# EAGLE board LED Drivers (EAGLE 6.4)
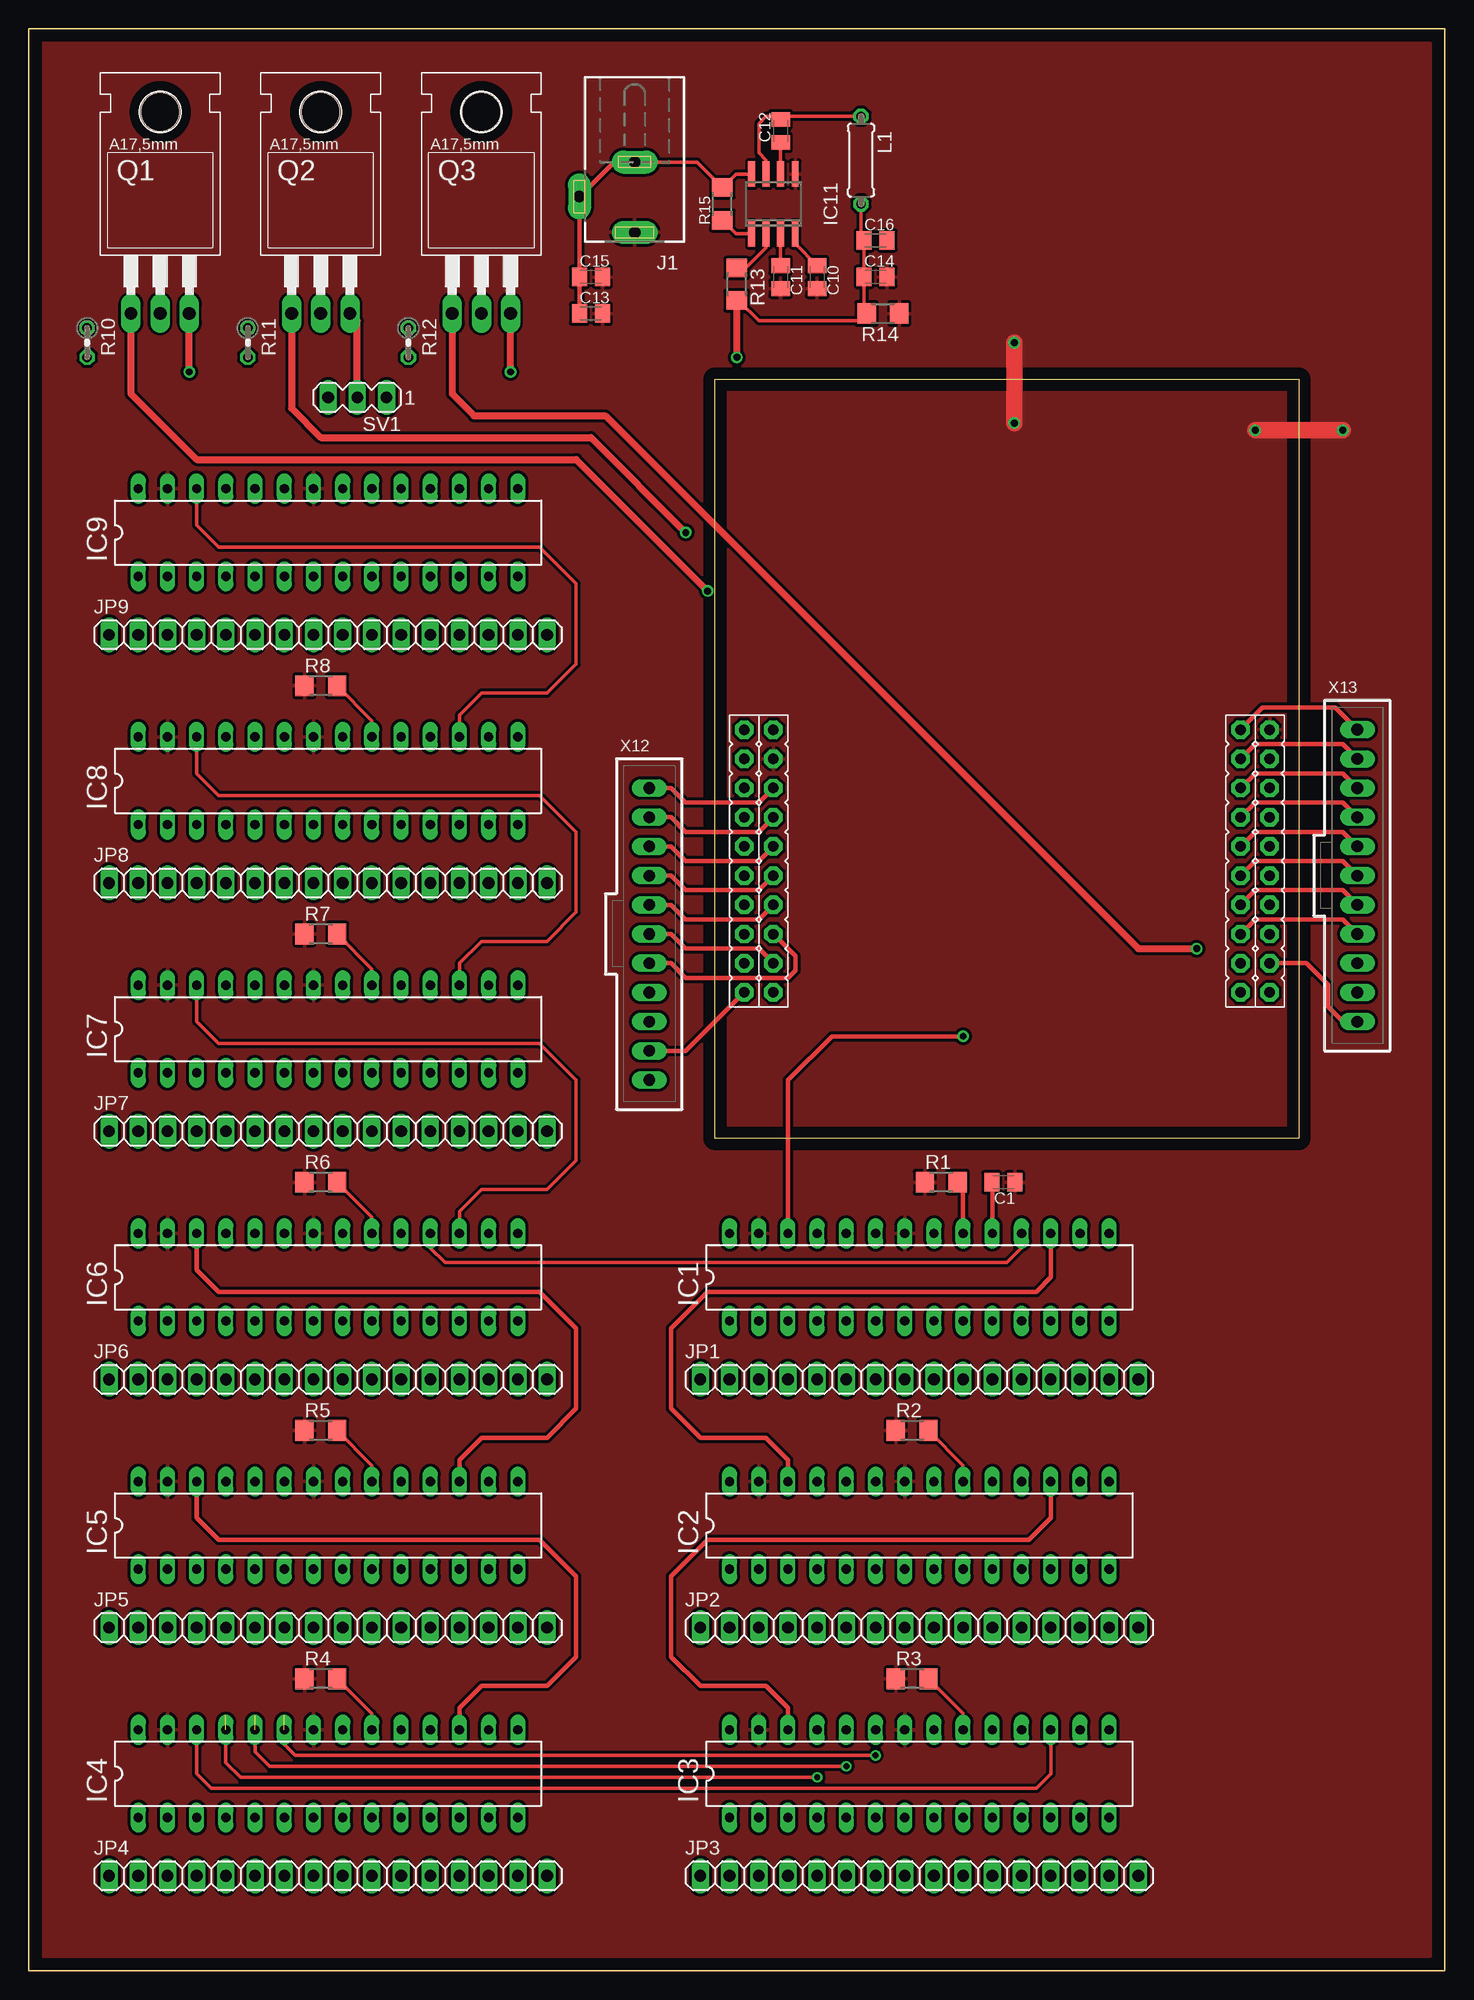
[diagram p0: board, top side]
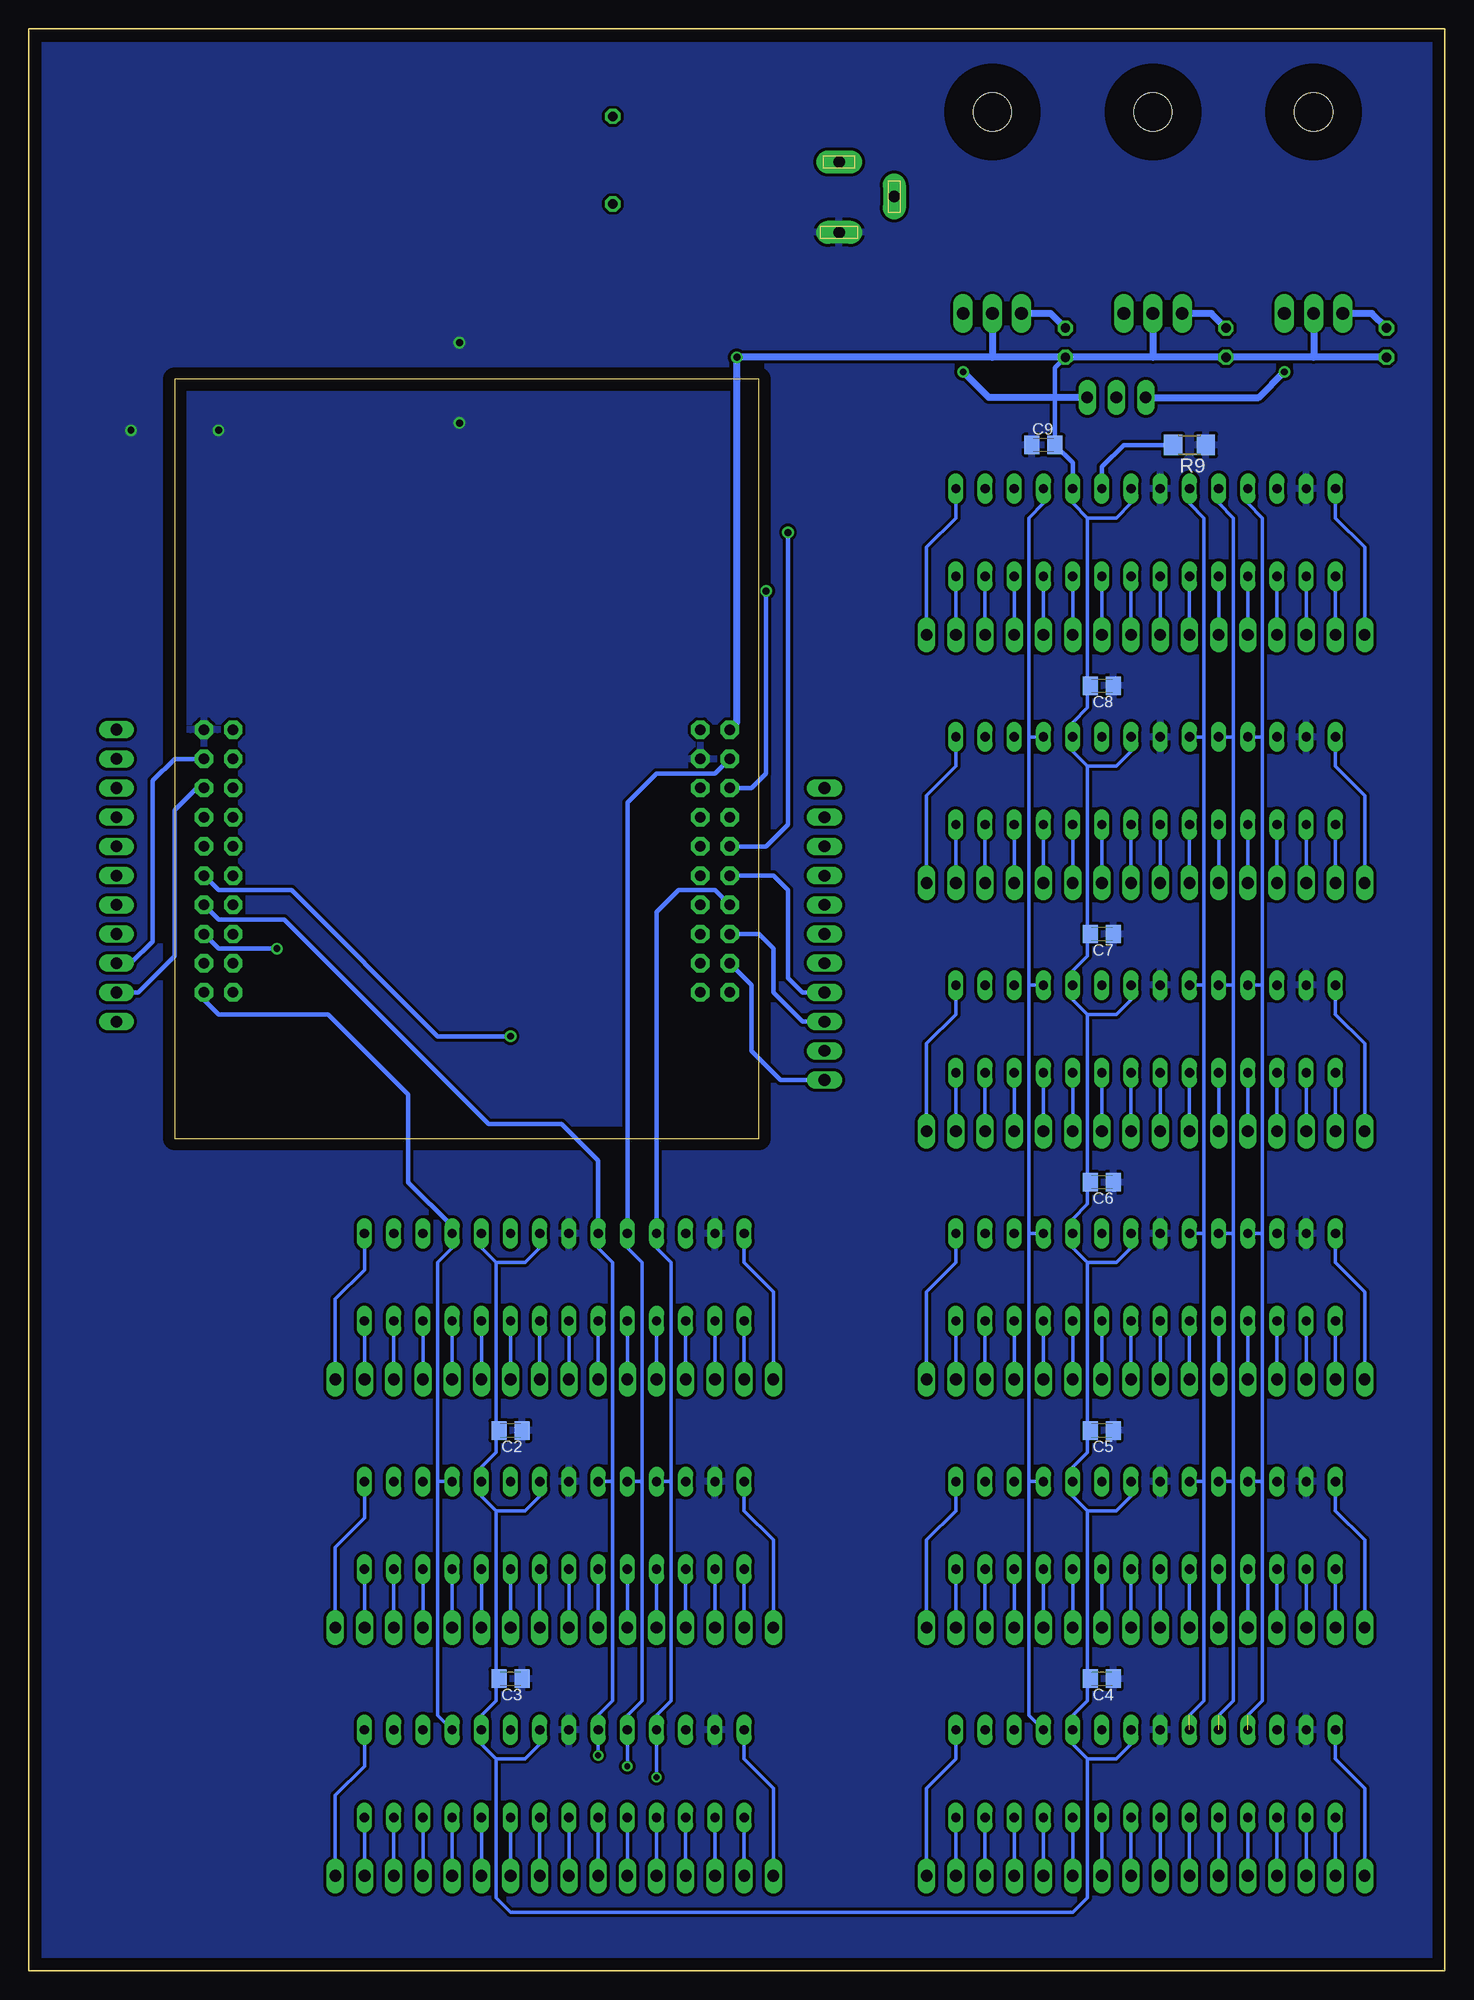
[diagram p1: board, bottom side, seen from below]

Size 123.19 x 168.91 mm. Coordinates in mm from the lower left corner, seen from the top.
Outline: 0,0 123.19,0 123.19,168.91 0,168.91 0,0
Copper layers (1*16): Top 0.035mm / dielectric 1.5mm / Bottom 0.035mm
Design rules "default *": minimum track width 10mil, minimum drill 24mil, track to track 10mil, track to pad 10mil, pad to pad 10mil, via to via 10mil, smd to smd 8mil, copper to edge 40mil, drill to drill 8mil, minimum pad ring 10mil, minimum via ring 8mil, stop-mask expansion 4mil, vias tented up to drill 0mil, thermal gap 10mil

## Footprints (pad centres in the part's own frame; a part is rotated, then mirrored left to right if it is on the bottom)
C0805K = smd 1.3 x 1.6: 1 -1,0; 2 1,0
DIP28 = drill 0.813 long: 1 -15.24,-3.81; 2 -12.7,-3.81; 3 -10.16,-3.81; 4 -7.62,-3.81; 5 -5.08,-3.81; 6 -2.54,-3.81; 7 0,-3.81; 8 2.54,-3.81; 9 5.08,-3.81; 10 7.62,-3.81; 11 10.16,-3.81; 12 12.7,-3.81; 13 15.24,-3.81; 14 17.78,-3.81; 15 17.78,3.81; 16 15.24,3.81; 17 12.7,3.81; 18 10.16,3.81; 19 7.62,3.81; 20 5.08,3.81; 21 2.54,3.81; 22 0,3.81; 23 -2.54,3.81; 24 -5.08,3.81; 25 -7.62,3.81; 26 -10.16,3.81; 27 -12.7,3.81; 28 -15.24,3.81
SOIC8 = smd 0.6 x 2.2: 1 -1.905,-2.6; 2 -0.635,-2.6; 3 0.635,-2.6; 4 1.905,-2.6; 5 1.905,2.6; 6 0.635,2.6; 7 -0.635,2.6; 8 -1.905,2.6
DCJ0202 = drill 1 pad 2 long: 1 0,3.1; 2 4.8,0; 3 0,-3
1X16 = drill 1.016 long: 1 -19.05,0; 2 -16.51,0; 3 -13.97,0; 4 -11.43,0; 5 -8.89,0; 6 -6.35,0; 7 -3.81,0; 8 -1.27,0; 9 1.27,0; 10 3.81,0; 11 6.35,0; 12 8.89,0; 13 11.43,0; 14 13.97,0; 15 16.51,0; 16 19.05,0
0207/7 = drill 0.813 octagon: 1 -3.81,0; 2 3.81,0
TO220 = drill 1.118 long: 1 -2.54,-6.35; 2 0,-6.35; 3 2.54,-6.35 | hole 3.302: 0,11.176
R1206 = smd 1.6 x 1.803: 1 -1.422,0; 2 1.422,0
0204V = drill 0.813 octagon: 1 -1.27,0; 2 1.27,0
MA03-1 = drill 1.016 long: 1 -2.54,0; 2 0,0; 3 2.54,0
LAUNCHPAD-XL = drill 0.914 pad 1.6 octagon: 3.3V 30.48,2.54; GND1 33.02,5.08; GND2 30.48,48.26; PA2 53.34,48.26; PA3 50.8,48.26; PA4 48.26,48.26; PA5 48.26,2.54; PA6 50.8,2.54; PA7 53.34,2.54; PB0 35.56,2.54; PB1 38.1,2.54; PB2 33.02,48.26; PB3 35.56,45.72; PB4 45.72,2.54; PB5 33.02,2.54; PB6 45.72,48.26; PB7 43.18,48.26; PC4 38.1,45.72; PC5 40.64,45.72; PC6 43.18,45.72; PC7 45.72,45.72; PD0 35.56,5.08; PD1 38.1,5.08; PD2 40.64,5.08; PD3 43.18,5.08; PD6 48.26,45.72; PD7 50.8,45.72; PE0 35.56,48.26; PE1 45.72,5.08; PE2 48.26,5.08; PE3 50.8,5.08; PE4 40.64,2.54; PE5 43.18,2.54; PF0 38.1,48.26; PF1 53.34,5.08; PF2 30.48,45.72; PF3 33.02,45.72; PF4 53.34,45.72; RST 40.64,48.26; VBUS 30.48,5.08
70543-11 = drill 1.016 long: 1 -12.7,0; 2 -10.16,0; 3 -7.62,0; 4 -5.08,0; 5 -2.54,0; 6 0,0; 7 2.54,0; 8 5.08,0; 9 7.62,0; 10 10.16,0; 11 12.7,0

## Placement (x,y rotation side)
C1  0.1uF  [C0805K]  84.77,68.58 180 top
C2  0.1uF  [C0805K]  81.28,46.99 180 bottom
C3  0.1uF  [C0805K]  81.28,25.4 180 bottom
C4  0.1uF  [C0805K]  29.84,25.4 180 bottom
C5  0.1uF  [C0805K]  29.84,46.99 180 bottom
C6  0.1uF  [C0805K]  29.84,68.58 180 bottom
C7  0.1uF  [C0805K]  29.84,90.17 180 bottom
C8  0.1uF  [C0805K]  29.84,111.76 180 bottom
C9  0.1uF  [C0805K]  34.92,132.72 0 bottom
C10  [C0805K]  68.58,147.32 270 top
C11  [C0805K]  65.41,147.32 270 top
C12  [C0805K]  65.41,160.02 90 top
C13  [C0805K]  48.9,144.15 0 top
C14  [C0805K]  73.66,147.32 0 top
C15  [C0805K]  48.9,147.32 0 top
C16  [C0805K]  73.66,150.5 0 top
IC1  [DIP28]  76.2,60.33 0 top
IC2  [DIP28]  76.2,38.73 0 top
IC3  [DIP28]  76.2,17.14 0 top
IC4  [DIP28]  24.77,17.14 0 top
IC5  [DIP28]  24.77,38.73 0 top
IC6  [DIP28]  24.77,60.33 0 top
IC7  [DIP28]  24.77,81.92 0 top
IC8  [DIP28]  24.77,103.5 0 top
IC9  [DIP28]  24.77,125.09 0 top
IC11  LT1257S  [SOIC8]  64.77,153.67 0 top
J1  DCJ0202  [DCJ0202]  52.7,154.31 180 top
JP1  [1X16]  77.47,51.44 0 top
JP2  [1X16]  77.47,29.84 0 top
JP3  [1X16]  77.47,8.26 0 top
JP4  [1X16]  26.04,8.26 0 top
JP5  [1X16]  26.04,29.84 0 top
JP6  [1X16]  26.04,51.44 0 top
JP7  [1X16]  26.04,73.03 0 top
JP8  [1X16]  26.04,94.61 0 top
JP9  [1X16]  26.04,116.2 0 top
L1  [0207/7]  72.39,157.48 270 top
Q1  BUZ171  [TO220]  11.43,150.5 0 top
Q2  BUZ171  [TO220]  25.4,150.5 0 top
Q3  BUZ171  [TO220]  39.37,150.5 0 top
R1  1.3K  [R1206]  79.38,68.58 0 top
R2  1.3K  [R1206]  76.83,46.99 0 top
R3  1.3K  [R1206]  76.83,25.4 0 top
R4  1.3K  [R1206]  25.4,25.4 0 top
R5  1.3K  [R1206]  25.4,46.99 0 top
R6  1.3K  [R1206]  25.4,68.58 0 top
R7  1.3K  [R1206]  25.4,90.17 0 top
R8  1.3K  [R1206]  25.4,111.76 0 top
R9  1.3K  [R1206]  22.23,132.72 180 bottom
R10  1K  [0204V]  5.08,141.6 270 top
R11  1K  [0204V]  19.05,141.6 270 top
R12  1K  [0204V]  33.02,141.6 270 top
R13  [R1206]  61.59,146.69 270 top
R14  [R1206]  74.3,144.15 180 top
R15  [R1206]  60.33,153.67 270 top
SV1  [MA03-1]  28.57,136.84 180 top
U$1  STELLARIS-LAUNCHPADSTELLARIS-LAUNCHPAD-XL  [LAUNCHPAD-XL]  59.69,138.43 270 top
X12  C-GRID-11-70543  [70543-11]  53.98,90.17 270 top
X13  C-GRID-11-70543  [70543-11]  115.57,95.25 270 top

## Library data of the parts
C1-C9 L1 = rcl
C10-C16 R1-R15 = resistor
IC1-IC9 = tcl5940(1)
IC11 = linear-technology; OC_FARNELL: unknown; OC_NEWARK: unknown
J1 = con-jack; OC_FARNELL: unknown; OC_NEWARK: unknown
JP1-JP9 = pinhead
Q1-Q3 = transistor-fet
SV1 = con-lstb; OC_FARNELL: unknown; OC_NEWARK: unknown
U$1 = StellarisLaunchPad_Fred
X12 X13 = con-molex; OC_FARNELL: unknown; OC_NEWARK: unknown

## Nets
+5V: C1.2 C2.2 C3.2 C4.2 C5.2 C6.2 C7.2 C8.2 C9.2 C14.1 C16.1 IC1.19 IC1.21 IC2.19 IC2.21 IC3.19 IC3.21 IC4.19 IC4.21 IC5.19 IC5.21 IC6.19 IC6.21 IC7.19 IC7.21 IC8.19 IC8.21 IC9.19 IC9.21 L1.2 Q1.2 Q2.2 Q3.2 R10.2 R11.2 R12.2 R13.2 R14.2 U$1.3.3V
GND: C1.1 C2.1 C3.1 C4.1 C5.1 C6.1 C7.1 C8.1 C9.1 C10.2 C11.2 C13.2 C14.2 C15.2 IC1.22 IC1.27 IC2.22 IC2.27 IC3.22 IC3.27 IC4.22 IC4.27 IC5.22 IC5.27 IC6.22 IC6.27 IC7.22 IC7.27 IC8.22 IC8.27 IC9.22 IC9.27 IC11.5 J1.1 R1.1 R2.1 R3.1 R4.1 R5.1 R6.1 R7.1 R8.1 R9.1 R14.1 U$1.GND1 U$1.GND2
N$1: IC1.17 IC2.26
N$2: IC1.20 R1.2
N$3: IC2.20 R2.2
N$4: IC2.28 JP2.1
N$5: IC2.3 JP2.4
N$6: IC2.4 JP2.5
N$7: IC2.5 JP2.6
N$8: IC2.6 JP2.7
N$9: IC2.7 JP2.8
N$10: IC2.8 JP2.9
N$11: IC2.9 JP2.10
N$12: IC2.10 JP2.11
N$13: IC2.11 JP2.12
N$14: IC2.12 JP2.13
N$15: IC1.28 JP1.1
N$16: IC2.13 JP2.14
N$17: IC2.14 JP2.15
N$18: IC2.15 JP2.16
N$19: IC1.1 JP1.2
N$20: IC1.2 JP1.3
N$21: IC1.3 JP1.4
N$22: IC1.4 JP1.5
N$23: IC1.5 JP1.6
N$24: IC1.6 JP1.7
N$25: IC1.7 JP1.8
N$26: IC1.8 JP1.9
N$27: IC1.9 JP1.10
N$28: IC1.10 JP1.11
N$29: IC1.11 JP1.12
N$30: IC1.12 JP1.13
N$31: IC1.13 JP1.14
N$32: IC1.14 JP1.15
N$33: IC1.15 JP1.16
N$34: IC2.1 JP2.2
N$35: IC2.2 JP2.3
N$36: IC2.17 IC3.26
N$37: IC3.20 R3.2
N$38: IC3.28 JP3.1
N$39: IC3.3 JP3.4
N$40: IC3.4 JP3.5
N$41: IC3.5 JP3.6
N$42: IC3.6 JP3.7
N$43: IC3.7 JP3.8
N$44: IC3.8 JP3.9
N$45: IC3.9 JP3.10
N$46: IC3.10 JP3.11
N$47: IC3.11 JP3.12
N$48: IC3.12 JP3.13
N$49: IC3.13 JP3.14
N$50: IC3.14 JP3.15
N$51: IC3.15 JP3.16
N$52: IC3.1 JP3.2
N$53: IC3.2 JP3.3
N$54: IC6.17 IC7.26
N$55: IC4.20 R4.2
N$56: IC4.28 JP4.1
N$57: IC4.3 JP4.4
N$58: IC4.4 JP4.5
N$59: IC4.5 JP4.6
N$60: IC4.6 JP4.7
N$61: IC4.7 JP4.8
N$62: IC4.8 JP4.9
N$63: IC4.9 JP4.10
N$64: IC4.10 JP4.11
N$65: IC4.11 JP4.12
N$66: IC4.12 JP4.13
N$67: IC4.13 JP4.14
N$68: IC4.14 JP4.15
N$69: IC4.15 JP4.16
N$70: IC4.1 JP4.2
N$71: IC4.2 JP4.3
N$72: IC4.17 IC5.26
N$73: IC5.20 R5.2
N$74: IC5.28 JP5.1
N$75: IC5.3 JP5.4
N$76: IC5.4 JP5.5
N$77: IC5.5 JP5.6
N$78: IC5.6 JP5.7
N$79: IC5.7 JP5.8
N$80: IC5.8 JP5.9
N$81: IC5.9 JP5.10
N$82: IC5.10 JP5.11
N$83: IC5.11 JP5.12
N$84: IC5.12 JP5.13
N$85: IC5.13 JP5.14
N$86: IC5.14 JP5.15
N$87: IC5.15 JP5.16
N$88: IC5.1 JP5.2
N$89: IC5.2 JP5.3
N$90: IC5.17 IC6.26
N$91: IC6.20 R6.2
N$92: IC6.28 JP6.1
N$93: IC6.3 JP6.4
N$94: IC6.4 JP6.5
N$95: IC6.5 JP6.6
N$96: IC6.6 JP6.7
N$97: IC6.7 JP6.8
N$98: IC6.8 JP6.9
N$99: IC6.9 JP6.10
N$100: IC6.10 JP6.11
N$101: IC6.11 JP6.12
N$102: IC6.12 JP6.13
N$103: IC6.13 JP6.14
N$104: IC6.14 JP6.15
N$105: IC6.15 JP6.16
N$106: IC6.1 JP6.2
N$107: IC6.2 JP6.3
N$108: IC1.25 IC2.25 IC3.25 IC4.25 IC5.25 IC6.25 IC7.25 IC8.25 IC9.25 U$1.PB4
N$109: IC7.20 R7.2
N$110: IC7.28 JP7.1
N$111: IC7.3 JP7.4
N$112: IC7.4 JP7.5
N$113: IC7.5 JP7.6
N$114: IC7.6 JP7.7
N$115: IC7.7 JP7.8
N$116: IC7.8 JP7.9
N$117: IC7.9 JP7.10
N$118: IC7.10 JP7.11
N$119: IC7.11 JP7.12
N$120: IC7.12 JP7.13
N$121: IC7.13 JP7.14
N$122: IC7.14 JP7.15
N$123: IC7.15 JP7.16
N$124: IC7.1 JP7.2
N$125: IC7.2 JP7.3
N$126: IC1.18 IC2.18 IC3.18 IC4.18 IC5.18 IC6.18 IC7.18 IC8.18 IC9.18 U$1.PA2
N$127: IC8.20 R8.2
N$128: IC8.28 JP8.1
N$129: IC8.3 JP8.4
N$130: IC8.4 JP8.5
N$131: IC8.5 JP8.6
N$132: IC8.6 JP8.7
N$133: IC8.7 JP8.8
N$134: IC8.8 JP8.9
N$135: IC8.9 JP8.10
N$136: IC8.10 JP8.11
N$137: IC8.11 JP8.12
N$138: IC8.12 JP8.13
N$139: IC8.13 JP8.14
N$140: IC8.14 JP8.15
N$141: IC8.15 JP8.16
N$142: IC8.1 JP8.2
N$143: IC8.2 JP8.3
N$144: IC8.17 IC9.26
N$145: IC9.20 R9.2
N$146: IC9.28 JP9.1
N$147: IC9.3 JP9.4
N$148: IC9.4 JP9.5
N$149: IC9.5 JP9.6
N$150: IC9.6 JP9.7
N$151: IC9.7 JP9.8
N$152: IC9.8 JP9.9
N$153: IC9.9 JP9.10
N$154: IC9.10 JP9.11
N$155: IC9.11 JP9.12
N$156: IC9.12 JP9.13
N$157: IC9.13 JP9.14
N$158: IC9.14 JP9.15
N$159: IC9.15 JP9.16
N$160: IC9.1 JP9.2
N$161: IC9.2 JP9.3
N$162: IC11.1 R15.2
N$163: IC1.26 U$1.PB7
N$164: U$1.PE1 X12.5
N$165: U$1.PF3 X13.2
N$166: U$1.PF2 X13.1
N$167: U$1.PB3 X13.3
N$168: U$1.PC4 X13.4
N$169: U$1.PC5 X13.5
N$170: U$1.PC6 X13.6
N$171: U$1.PC7 X13.7
N$172: U$1.PD6 X13.8
N$173: U$1.PB2 X13.9
N$174: U$1.PE0 X13.10
N$175: U$1.PA3 X13.11
N$176: Q3.1 R12.1 U$1.PA4
N$177: Q2.1 R11.1 U$1.PE4
N$178: U$1.PD0 X12.1
N$179: U$1.PD1 X12.2
N$180: U$1.PD2 X12.3
N$181: U$1.PD3 X12.4
N$182: IC1.23 IC2.23 IC3.23 IC4.23 IC5.23 IC6.23 IC7.23 IC8.23 IC9.23 U$1.PB6
N$183: U$1.PE3 X12.6
N$184: U$1.PE2 X12.7
N$185: U$1.PE5 X12.8
N$186: U$1.PA5 X12.9
N$187: U$1.PA7 X12.10
N$188: U$1.PA6 X12.11
N$189: IC1.24 IC2.24 IC3.24 IC4.24 IC5.24 IC6.24 IC7.24 IC8.24 IC9.24 U$1.PB5
N$190: Q1.3 SV1.3
N$191: Q2.3 SV1.2
N$192: Q3.3 SV1.1
N$193: Q1.1 R10.1 U$1.PB0
N$194: C13.1 C15.1 IC11.8 J1.2 J1.3 R15.1
N$195: C11.1 IC11.3
N$197: C10.1 IC11.4
N$198: C12.1 IC11.6
N$199: C12.2 IC11.7 L1.1
N$200: IC11.2 R13.1
N$202: IC3.17 IC4.26
N$204: IC7.17 IC8.26
RST: U$1.RST
VBUS: U$1.VBUS

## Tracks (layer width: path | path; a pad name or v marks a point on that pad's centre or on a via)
+5V  (via drill 0.6)
  Top 0.305: L1.2 72.39,150.76 C16.1 C14.1 72.66,144.36 R14.2 72.24,143.51 63.5,143.51 61.75,145.26 R13.2 61.59,144.78
  Top 0.406: IC1.19 83.82,68.53 C1.2
  Top 0.61: v61.59,140.34 R13.2
  Bottom 0.305: IC4.21 27.3,19.68 28.57,18.41 31.11,18.41 | 31.11,126.36 32.38,127.64 IC9.19 | IC9.21 27.3,127.64 28.57,126.36 31.11,126.36 | 31.11,104.78 32.38,106.05 IC8.19 32.38,108.58 31.11,109.86 31.11,111.49 C8.2 31.11,112.03 31.11,126.36 | IC8.21 27.3,106.05 28.57,104.78 31.11,104.78 | 31.11,83.19 32.38,84.45 IC7.19 32.38,87 31.11,88.27 31.11,89.9 C7.2 31.11,90.44 31.11,104.78 | IC7.21 27.3,84.45 28.57,83.19 31.11,83.19 | 31.11,61.59 32.38,62.87 IC6.19 32.38,65.41 31.11,66.67 31.11,68.31 C6.2 31.11,68.85 31.11,83.19 | IC6.21 27.3,62.87 28.57,61.59 31.11,61.59 | 31.11,40.01 32.38,41.27 IC5.19 32.38,43.81 31.11,45.09 31.11,46.62 | 31.11,18.41 32.38,19.68 IC4.19 32.38,22.23 31.11,23.5 31.11,25.13 C4.2 31.11,25.67 31.11,40.01 | IC5.21 27.3,41.27 28.57,40.01 31.11,40.01 | IC3.21 78.74,19.68 80.01,18.41 82.55,18.41 | 82.55,40.01 83.82,41.27 IC2.19 83.82,43.81 82.55,45.09 82.55,46.72 | IC2.21 78.74,41.27 80.01,40.01 82.55,40.01 | 82.55,61.59 83.82,62.87 IC1.19 | IC1.21 78.74,62.87 80.01,61.59 82.55,61.59 | 82.55,18.41 83.82,19.68 IC3.19 83.82,22.23 82.55,23.5 82.55,25.13 C3.2 82.55,25.67 82.55,40.01 | 82.55,18.41 82.55,6.35 81.28,5.08 32.38,5.08 31.11,6.35 31.11,18.41 | 82.55,46.72 C2.2 | 82.55,61.59 82.55,46.72 | 31.11,46.72 C5.2 31.11,46.62 | 31.11,61.59 31.11,46.72 | 31.11,46.72 31.11,46.62
  Bottom 0.406: IC9.19 32.38,131.18 C9.2 33.92,139.43 R12.2
  Bottom 0.61: R10.2 11.43,140.34 | 11.43,140.34 R11.2 25.4,140.34 | 25.4,140.34 R12.2 39.37,140.34 | Q1.2 11.43,140.34 | Q2.2 25.4,140.34 | 39.37,140.34 v61.59,140.34 61.59,108.58 U$1.3.3V | Q3.2 39.37,140.34
GND  (via drill 0.6)
  Top 1.422: v85.72,141.6 v85.72,134.62 | v114.3,133.99 v106.68,133.99
  pour Bottom: 1.27,1.27 121.92,1.27 121.92,167.64 1.27,167.64
  pour Top: 1.27,1.27 121.92,1.27 121.92,167.64 1.27,167.64
N$1
  Top 0.406: IC1.17 88.9,60.33 87.63,59.05 59.05,59.05 55.88,55.88 55.88,48.9 58.42,46.35 64.14,46.35 66.04,44.45 IC2.26
N$2
  Top 0.406: IC1.20 81.28,68.1 R1.2
N$3
  Top 0.305: IC2.20 81.28,43.97 R2.2
N$4
  Bottom 0.305: IC2.28 60.96,40.01 58.42,37.47 JP2.1
N$5
  Bottom 0.305: IC2.3 JP2.4
N$6
  Bottom 0.305: IC2.4 JP2.5
N$7
  Bottom 0.305: IC2.5 JP2.6
N$8
  Bottom 0.305: IC2.6 JP2.7
N$9
  Bottom 0.305: IC2.7 JP2.8
N$10
  Bottom 0.305: JP2.9 IC2.8
N$11
  Bottom 0.305: IC2.9 JP2.10
N$12
  Bottom 0.305: IC2.10 JP2.11
N$13
  Bottom 0.305: IC2.11 JP2.12
N$14
  Bottom 0.305: IC2.12 JP2.13
N$15
  Bottom 0.305: IC1.28 60.96,61.59 58.42,59.05 JP1.1
N$16
  Bottom 0.305: IC2.13 JP2.14
N$17
  Bottom 0.305: IC2.14 JP2.15
N$18
  Bottom 0.305: IC2.15 93.98,39.37 96.52,36.83 JP2.16
N$19
  Bottom 0.305: IC1.1 JP1.2
N$20
  Bottom 0.305: IC1.2 JP1.3
N$21
  Bottom 0.305: IC1.3 JP1.4
N$22
  Bottom 0.305: IC1.4 JP1.5
N$23
  Bottom 0.305: IC1.5 JP1.6
N$24
  Bottom 0.305: IC1.6 JP1.7
N$25
  Bottom 0.305: IC1.7 JP1.8
N$26
  Bottom 0.305: IC1.8 JP1.9
N$27
  Bottom 0.305: IC1.9 JP1.10
N$28
  Bottom 0.305: IC1.10 JP1.11
N$29
  Bottom 0.305: IC1.11 JP1.12
N$30
  Bottom 0.305: IC1.12 JP1.13
N$31
  Bottom 0.305: IC1.13 JP1.14
N$32
  Bottom 0.305: IC1.14 JP1.15
N$33
  Bottom 0.305: IC1.15 93.98,60.96 96.52,58.42 JP1.16
N$34
  Bottom 0.305: IC2.1 JP2.2
N$35
  Bottom 0.305: JP2.3 IC2.2
N$36
  Top 0.406: IC2.17 88.9,39.37 87,37.47 59.05,37.47 55.88,34.29 55.88,27.3 58.42,24.77 64.14,24.77 66.04,22.86 IC3.26
N$37
  Top 0.305: IC3.20 81.28,22.38 R3.2
N$38
  Bottom 0.305: IC3.28 60.96,18.41 58.42,15.88 JP3.1
N$39
  Bottom 0.305: IC3.3 JP3.4
N$40
  Bottom 0.305: IC3.4 JP3.5
N$41
  Bottom 0.305: IC3.5 JP3.6
N$42
  Bottom 0.305: IC3.6 JP3.7
N$43
  Bottom 0.305: IC3.7 JP3.8
N$44
  Bottom 0.305: IC3.8 JP3.9
N$45
  Bottom 0.305: IC3.9 JP3.10
N$46
  Bottom 0.305: IC3.10 JP3.11
N$47
  Bottom 0.305: IC3.11 JP3.12
N$48
  Bottom 0.305: IC3.12 JP3.13
N$49
  Bottom 0.305: IC3.13 JP3.14
N$50
  Bottom 0.305: IC3.14 JP3.15
N$51
  Bottom 0.305: IC3.15 93.98,17.78 96.52,15.24 JP3.16
N$52
  Bottom 0.305: IC3.1 JP3.2
N$53
  Bottom 0.305: IC3.2 JP3.3
N$54
  Top 0.305: IC6.17 37.47,66.04 39.37,67.94 45.09,67.94 47.62,70.48 47.62,77.47 44.45,80.64 16.51,80.64 14.61,82.55 IC7.26
N$55
  Top 0.305: IC4.20 29.84,22.38 R4.2
N$56
  Bottom 0.305: JP4.1 6.99,15.88 9.53,18.41 IC4.28
N$57
  Bottom 0.305: JP4.4 IC4.3
N$58
  Bottom 0.305: IC4.4 JP4.5
N$59
  Bottom 0.305: JP4.6 IC4.5
N$60
  Bottom 0.305: IC4.6 JP4.7
N$61
  Bottom 0.305: JP4.8 IC4.7
N$62
  Bottom 0.305: IC4.8 JP4.9
N$63
  Bottom 0.305: JP4.10 IC4.9
N$64
  Bottom 0.305: IC4.10 JP4.11
N$65
  Bottom 0.305: JP4.12 IC4.11
N$66
  Bottom 0.305: IC4.12 JP4.13
N$67
  Bottom 0.305: JP4.14 IC4.13
N$68
  Bottom 0.305: IC4.14 JP4.15
N$69
  Bottom 0.305: IC4.15 42.55,18.41 45.09,15.88 JP4.16
N$70
  Bottom 0.305: JP4.2 IC4.1
N$71
  Bottom 0.305: IC4.2 JP4.3
N$72
  Top 0.406: IC4.17 37.47,22.86 39.37,24.77 45.09,24.77 47.62,27.3 47.62,34.29 44.45,37.47 16.51,37.47 14.61,39.37 IC5.26
N$73
  Top 0.305: IC5.20 29.84,43.97 R5.2
N$74
  Bottom 0.305: IC5.28 9.53,40.01 6.99,37.47 JP5.1
N$75
  Bottom 0.305: JP5.4 IC5.3
N$76
  Bottom 0.305: JP5.5 IC5.4
N$77
  Bottom 0.305: IC5.5 JP5.6
N$78
  Bottom 0.305: JP5.7 IC5.6
N$79
  Bottom 0.305: IC5.7 JP5.8
N$80
  Bottom 0.305: JP5.9 IC5.8
N$81
  Bottom 0.305: IC5.9 JP5.10
N$82
  Bottom 0.305: JP5.11 IC5.10
N$83
  Bottom 0.305: IC5.11 JP5.12
N$84
  Bottom 0.305: JP5.13 IC5.12
N$85
  Bottom 0.305: IC5.13 JP5.14
N$86
  Bottom 0.305: JP5.15 IC5.14
N$87
  Bottom 0.305: IC5.15 42.55,40.01 45.09,37.47 JP5.16
N$88
  Bottom 0.305: JP5.2 IC5.1
N$89
  Bottom 0.305: IC5.2 JP5.3
N$90
  Top 0.406: IC5.17 37.47,44.45 39.37,46.35 45.09,46.35 47.62,48.9 47.62,55.88 44.45,59.05 16.51,59.05 14.61,60.96 IC6.26
N$91
  Top 0.305: IC6.20 29.84,65.56 R6.2
N$92
  Bottom 0.305: IC6.28 9.53,61.59 6.99,59.05 JP6.1
N$93
  Bottom 0.305: IC6.3 JP6.4
N$94
  Bottom 0.305: IC6.4 JP6.5
N$95
  Bottom 0.305: IC6.5 JP6.6
N$96
  Bottom 0.305: IC6.6 JP6.7
N$97
  Bottom 0.305: IC6.7 JP6.8
N$98
  Bottom 0.305: IC6.8 JP6.9
N$99
  Bottom 0.305: IC6.9 JP6.10
N$100
  Bottom 0.305: IC6.10 JP6.11
N$101
  Bottom 0.305: IC6.11 JP6.12
N$102
  Bottom 0.305: JP6.13 IC6.12
N$103
  Bottom 0.305: IC6.13 JP6.14
N$104
  Bottom 0.305: JP6.15 IC6.14
N$105
  Bottom 0.305: IC6.15 42.55,61.59 45.09,59.05 JP6.16
N$106
  Bottom 0.305: IC6.1 JP6.2
N$107
  Bottom 0.305: IC6.2 JP6.3
N$108  (via drill 0.5)  (1 unrouted)
  Top 0.305: IC4.25 17.14,18.1 18.41,16.83 v68.58,16.83
  Bottom 0.305: 17.14,22.23 15.88,23.5 15.88,42.55 | 15.88,42.55 15.88,64.14 | 15.88,64.14 15.88,85.72 | 15.88,85.72 15.88,107.31 | 15.88,107.31 15.88,126.36 17.14,127.64 IC9.25 | IC8.25 15.88,107.31 | IC6.25 15.88,64.14 | IC5.25 15.88,42.55 | IC1.25 68.58,62.87 67.31,61.59 67.31,42.55 | 67.31,42.55 67.31,23.5 68.58,22.23 IC3.25 v68.58,16.83 | IC2.25 67.31,42.55 | IC7.25 15.88,85.72
  Bottom 0.406: IC1.25 68.58,92.08 66.67,93.98 63.5,93.98 U$1.PB4
N$109
  Top 0.305: IC7.20 29.84,87.15 R7.2
N$110
  Bottom 0.305: JP7.1 6.99,80.64 9.53,83.19 IC7.28
N$111
  Bottom 0.305: IC7.3 JP7.4
N$112
  Bottom 0.305: IC7.4 JP7.5
N$113
  Bottom 0.305: IC7.5 JP7.6
N$114
  Bottom 0.305: IC7.6 JP7.7
N$115
  Bottom 0.305: IC7.7 JP7.8
N$116
  Bottom 0.305: JP7.9 IC7.8
N$117
  Bottom 0.305: IC7.9 JP7.10
N$118
  Bottom 0.305: JP7.11 IC7.10
N$119
  Bottom 0.305: JP7.12 IC7.11
N$120
  Bottom 0.305: JP7.13 IC7.12
N$121
  Bottom 0.305: JP7.14 IC7.13
N$122
  Bottom 0.305: JP7.15 IC7.14
N$123
  Bottom 0.305: IC7.15 42.55,83.19 45.09,80.64 JP7.16
N$124
  Bottom 0.305: JP7.2 IC7.1
N$125
  Bottom 0.305: IC7.2 JP7.3
N$126
  Top 0.305: IC1.18 86.36,62.87 85.09,61.59 36.2,61.59 34.92,62.87 IC6.18
  Bottom 0.305: IC1.18 86.36,62.87 87.63,61.59 87.63,42.55 | 87.63,42.55 87.63,22.23 IC3.18 | IC2.18 87.63,42.55 | IC4.18 36.2,22.23 36.2,42.55 | 36.2,42.55 36.2,64.14 | 36.2,64.14 36.2,85.72 | 36.2,85.72 IC7.18 | IC6.18 36.2,64.14 | IC5.18 36.2,42.55 | IC9.18 34.92,127.64 36.2,126.36 36.2,107.31 | 36.2,107.31 36.2,85.72 | IC8.18 36.2,107.31
  Bottom 0.406: U$1.PA2 107.95,84.45 106.68,83.19 97.16,83.19 90.17,76.2 90.17,68.58 86.36,64.77 IC1.18
N$127
  Top 0.305: IC8.20 29.84,108.74 R8.2
N$128
  Bottom 0.305: IC8.28 9.53,104.78 6.99,102.23 JP8.1
N$129
  Bottom 0.305: IC8.3 JP8.4
N$130
  Bottom 0.305: IC8.4 JP8.5
N$131
  Bottom 0.305: IC8.5 JP8.6
N$132
  Bottom 0.305: JP8.7 IC8.6
N$133
  Bottom 0.305: JP8.8 IC8.7
N$134
  Bottom 0.305: IC8.8 JP8.9
N$135
  Bottom 0.305: JP8.10 IC8.9
N$136
  Bottom 0.305: IC8.10 JP8.11
N$137
  Bottom 0.305: JP8.12 IC8.11
N$138
  Bottom 0.305: IC8.12 JP8.13
N$139
  Bottom 0.305: JP8.14 IC8.13
N$140
  Bottom 0.305: IC8.14 JP8.15
N$141
  Bottom 0.305: IC8.15 42.55,104.78 45.09,102.23 JP8.16
N$142
  Bottom 0.305: JP8.2 IC8.1
N$143
  Bottom 0.305: JP8.3 IC8.2
N$144
  Top 0.305: IC8.17 37.47,109.22 39.37,111.12 45.09,111.12 47.62,113.67 47.62,120.65 44.45,123.83 16.51,123.83 14.61,125.73 IC9.26
N$145
  Bottom 0.406: IC9.20 29.84,130.81 27.94,132.72 R9.2
N$146
  Bottom 0.305: IC9.28 9.53,126.36 6.99,123.83 JP9.1
N$147
  Bottom 0.305: JP9.4 IC9.3
N$148
  Bottom 0.305: IC9.4 JP9.5
N$149
  Bottom 0.305: JP9.6 IC9.5
N$150
  Bottom 0.305: IC9.6 JP9.7
N$151
  Bottom 0.305: JP9.8 IC9.7
N$152
  Bottom 0.305: IC9.8 JP9.9
N$153
  Bottom 0.305: JP9.10 IC9.9
N$154
  Bottom 0.305: IC9.10 JP9.11
N$155
  Bottom 0.305: JP9.12 IC9.11
N$156
  Bottom 0.305: IC9.12 JP9.13
N$157
  Bottom 0.305: JP9.14 IC9.13
N$158
  Bottom 0.305: IC9.14 JP9.15
N$159
  Bottom 0.305: IC9.15 42.55,126.36 45.09,123.83 JP9.16
N$160
  Bottom 0.305: JP9.2 IC9.1
N$161
  Bottom 0.305: IC9.2 JP9.3
N$162
  Top 0.305: IC11.1 61.5,151.07 R15.2
N$163  (via drill 0.6)
  Top 0.406: IC1.26 66.04,77.47 69.85,81.28 v81.28,81.28
  Bottom 0.406: U$1.PB7 106.68,93.98 100.33,93.98 87.63,81.28 v81.28,81.28
N$164
  Top 0.406: U$1.PE1 63.5,91.44 57.15,91.44 55.88,92.71 X12.5
N$165
  Top 0.406: U$1.PF3 106.68,106.68 114.3,106.68 X13.2
N$166
  Top 0.406: U$1.PF2 107.31,109.86 113.67,109.86 X13.1
N$167
  Top 0.406: U$1.PB3 106.68,104.14 114.3,104.14 X13.3
N$168
  Top 0.406: U$1.PC4 106.68,101.6 114.3,101.6 X13.4
N$169
  Top 0.406: U$1.PC5 106.68,99.06 114.3,99.06 X13.5
N$170
  Top 0.406: U$1.PC6 106.68,96.52 114.3,96.52 X13.6
N$171
  Top 0.406: U$1.PC7 106.68,93.98 114.3,93.98 X13.7
N$172
  Top 0.406: U$1.PD6 106.68,91.44 114.3,91.44 X13.8
N$173
  Bottom 0.406: X13.9 114.3,87.63 112.39,89.53 112.39,103.5 110.49,105.41 U$1.PB2
N$174
  Bottom 0.406: U$1.PE0 108.58,102.87 110.49,100.97 110.49,88.27 113.67,85.09 X13.10
N$175
  Top 0.406: X13.11 114.3,82.55 113.03,83.82 113.03,85.72 111.12,87.63 U$1.PA3
N$176  (via drill 0.6)
  Top 0.61: Q3.1 36.83,137.16 38.73,135.25 50.16,135.25 96.52,88.9 v101.6,88.9
  Bottom 0.406: U$1.PA4 106.68,88.9 v101.6,88.9
  Bottom 0.61: R12.1 34.29,144.15 Q3.1
N$177  (via drill 0.6)
  Top 0.61: Q2.1 22.86,135.89 25.4,133.35 48.9,133.35 v57.15,125.09
  Bottom 0.406: v57.15,125.09 57.15,99.69 59.05,97.79 U$1.PE4
  Bottom 0.61: R11.1 20.32,144.15 Q2.1
N$178
  Top 0.406: U$1.PD0 63.5,101.6 57.15,101.6 55.88,102.87 X12.1
N$179
  Top 0.406: U$1.PD1 63.5,99.06 57.15,99.06 55.88,100.33 X12.2
N$180
  Top 0.406: U$1.PD2 63.5,96.52 57.15,96.52 55.88,97.79 X12.3
N$181
  Top 0.406: U$1.PD3 63.5,93.98 57.15,93.98 55.88,95.25 X12.4
N$182  (via drill 0.5)  (1 unrouted)
  Top 0.305: IC4.23 22.23,19.68 23.18,18.73 v73.66,18.73
  Bottom 0.305: 22.23,22.23 20.95,23.5 20.95,42.55 | 20.95,42.55 20.95,64.14 | 20.95,64.14 20.95,85.72 | 20.95,85.72 20.95,107.31 | 20.95,107.31 20.95,126.36 22.23,127.64 IC9.23 | IC8.23 20.95,107.31 | IC7.23 20.95,85.72 | IC6.23 20.95,64.14 | IC5.23 20.95,42.55 | IC1.23 73.66,62.87 72.39,61.59 72.39,42.55 | 72.39,42.55 72.39,23.5 73.66,22.23 IC3.23 v73.66,18.73 | IC2.23 72.39,42.55
  Bottom 0.406: U$1.PB6 106.68,91.44 100.97,91.44 83.19,73.66 76.83,73.66 73.66,70.48 IC1.23
N$183
  Top 0.406: X12.6 55.88,90.17 57.15,88.9 63.5,88.9 U$1.PE3
N$184
  Top 0.406: U$1.PE2 66.67,88.27 66.67,87 66.04,86.36 57.15,86.36 55.88,87.63 X12.7
N$185
  Bottom 0.406: X12.8 55.88,85.09 57.15,86.36 57.15,93.98 58.42,95.25 U$1.PE5
N$186
  Bottom 0.406: X12.9 55.88,82.55 58.42,85.09 58.42,88.9 59.69,90.17 U$1.PA5
N$187
  Top 0.406: X12.10 57.15,80.01 U$1.PA7
N$188
  Bottom 0.406: X12.11 57.78,77.47 60.33,80.01 60.33,85.72 U$1.PA6
N$189  (via drill 0.5)  (1 unrouted)
  Top 0.305: IC4.24 19.68,19.05 20.95,17.78 v71.12,17.78
  Bottom 0.305: IC9.24 19.68,127.64 18.41,126.36 18.41,107.31 | 18.41,107.31 18.41,85.72 | 18.41,85.72 18.41,64.14 | 18.41,64.14 18.41,42.55 | 18.41,42.55 18.41,23.5 19.68,22.23 | IC8.24 18.41,107.31 | IC7.24 18.41,85.72 | IC6.24 18.41,64.14 | IC5.24 18.41,42.55 | 69.85,42.55 69.85,23.5 71.12,22.23 IC3.24 v71.12,17.78 | 69.85,42.55 69.85,61.59 71.12,62.87 IC1.24 | IC2.24 69.85,42.55
  Bottom 0.406: IC1.24 71.12,101.6 68.58,104.14 63.5,104.14 U$1.PB5
N$190  (via drill 0.6)
  Top 0.61: v13.97,139.06 Q1.3
  Bottom 0.61: SV1.3 16.19,136.84 v13.97,139.06
N$191
  Top 0.61: SV1.2 28.57,143.51 Q2.3
N$192  (via drill 0.6)
  Top 0.61: v41.91,139.06 Q3.3
  Bottom 0.61: SV1.1 39.69,136.84 v41.91,139.06
N$193  (via drill 0.6)
  Top 0.61: Q1.1 8.89,137.16 14.61,131.44 47.62,131.44 v59.05,120.02
  Bottom 0.406: U$1.PB0 60.33,102.87 59.05,104.14 v59.05,120.02
  Bottom 0.61: R10.1 6.35,144.15 Q1.1
N$194
  Top 0.305: IC11.8 61.5,156.27 R15.1 58.11,157.31 J1.3
  Top 0.406: J1.3 50.91,157.31 J1.2 C15.1 | C15.1 C13.1
  Top 0.61: C15.1
N$195
  Top 0.305: IC11.3 C11.1
N$197
  Top 0.305: IC11.4 66.67,150.22 C10.1
N$198
  Top 0.305: IC11.6 C12.1
N$199
  Top 0.305: IC11.7 64.14,157.48 63.5,158.12 63.5,160.66 64.14,161.29 65.14,161.29 C12.2 65.67,161.29 L1.1
N$200
  Top 0.305: IC11.2 64.14,149.86 62.23,147.96 61.75,147.96 R13.1
N$202
  Top 0.305: IC3.17 88.9,17.14 87.63,15.88 15.88,15.88 14.61,17.14 IC4.26
N$204
  Top 0.305: IC7.17 37.47,87.63 39.37,89.53 45.09,89.53 47.62,92.08 47.62,99.06 44.45,102.23 16.51,102.23 14.61,104.14 IC8.26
